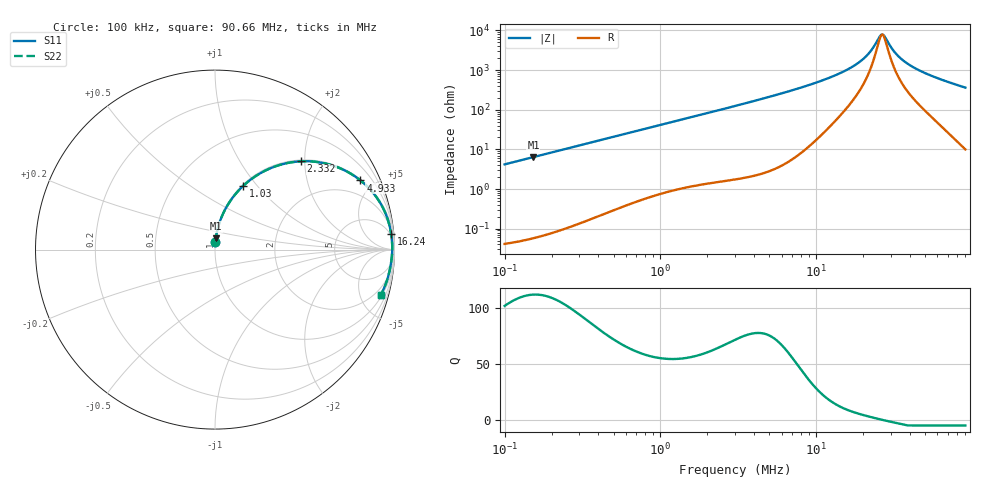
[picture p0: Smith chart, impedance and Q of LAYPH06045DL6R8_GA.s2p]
! LAYPH06045DL6R8_GA  S-PARAMETER MODEL  ( General Type )
! Model Generated by TAIYO YUDEN Corporation (http://www.ty-top.com)
! Version 2.0
! TAIYO YUDEN Control No. 180914NI43SB-FBB
! Copyright(c) 2018 TAIYO YUDEN CO.,LTD. All Rights Reserved.
! Product Description (link to TY-COMPAS)
! https://ds.yuden.co.jp/TYCOMPAS/or/detail?pn=LAYPH06045DL6R8NGA&u=M
! Products Name : Inductors
! Characteristics :
!  Inductance : 6.8 uH , SRF(min) : -Hz , DC Resistance(max) : 0.0377 Ohm
!  Rated Current : Saturation :2.5 A , Temp Rise : 2 A (25 degC)
!  Case Size : 6.3 x 6.0 / 0.248 x 0.236 [mm/inch] , Thickness : 4.5 / 0.177 [mm/inch]
!  (Conditions: Temperature = 25 degC , DC Bias Current/Voltage = 0A / 0V)
! External Node Assignments :
!  1  o---GGG---o  2
! GND o---------o GND
! Frequency Range : 0.1MHz  -  90.659724MHz  [ 402 STEP ]
# MHz S RI R 50
! Freq[MHz].  S11 Real  S11 Imag  S21 Real  S21 Imag  S12 Real  S12 Imag  S22 Real  S22 Imag
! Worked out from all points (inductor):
!   401 points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, 100 kHz to 90.66 MHz, reference 50 ohm
!   read as one part in series: L = 6.67 uH near 103.5 kHz
!   highest Q = 112 at 153.1 kHz (marker M1), where L = 6.67 uH
!   self-resonance near 26.16 MHz
!   S11 on the Smith chart (normalised r, x): 100 kHz: 1.00, +0.08; 1.03 MHz: 1.02, +0.85; 2.332 MHz: 1.03, +1.92; 4.933 MHz: 1.06, +4.18; 16.24 MHz: 4, +22; 90.66 MHz: 1.20, -7.24
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0.1  0.00216 0.0418  0.9978 -0.0418  0.9978 -0.0418  0.00216 0.0418
0.153052  0.00466 0.0638  0.9953 -0.0638  0.9953 -0.0638  0.00466 0.0638
0.312872  0.0182 0.1283  0.9818 -0.1283  0.9818 -0.1283  0.0182 0.1283
0.597477  0.0614 0.2326  0.9386 -0.2326  0.9386 -0.2326  0.0614 0.2326
0.97889  0.1455 0.3436  0.8545 -0.3436  0.8545 -0.3436  0.1455 0.3436
1.030183  0.1582 0.3559  0.8418 -0.3559  0.8418 -0.3559  0.1582 0.3559
1.523933  0.286 0.443  0.714 -0.443  0.714 -0.443  0.286 0.443
2.332406  0.4799 0.4918  0.5201 -0.4918  0.5201 -0.4918  0.4799 0.4918
3.062674  0.6143 0.4799  0.3857 -0.4799  0.3857 -0.4799  0.6143 0.4799
4.933098  0.8104 0.3854  0.1896 -0.3854  0.1896 -0.3854  0.8104 0.3854
9.420503  0.9465 0.2099  0.0535 -0.2099  0.0535 -0.2099  0.9465 0.2099
12.79846  0.9714 0.1374  0.0286 -0.1374  0.0286 -0.1374  0.9714 0.1374
16.24304  0.9812 0.0885  0.0188 -0.0885  0.0188 -0.0885  0.9812 0.0885
18.61296  0.9845 0.063  0.0155 -0.063  0.0155 -0.063  0.9845 0.063
20.96864  0.9864 0.0414  0.0136 -0.0414  0.0136 -0.0414  0.9864 0.0414
26.16292  0.9876 0.00253  0.0124 -0.00253  0.0124 -0.00253  0.9876 0.00253
27.53385  0.9874 -0.00635  0.0126 0.00635  0.0126 0.00635  0.9874 -0.00635
29.47413  0.9869 -0.0182  0.0131 0.0182  0.0131 0.0182  0.9869 -0.0182
34.35444  0.9847 -0.0449  0.0153 0.0449  0.0153 0.0449  0.9847 -0.0449
42.14104  0.9797 -0.0813  0.0203 0.0813  0.0203 0.0813  0.9797 -0.0813
58.23478  0.9662 -0.1449  0.0338 0.1449  0.0338 0.1449  0.9662 -0.1449
90.65972  0.9232 -0.2529  0.0768 0.2529  0.0768 0.2529  0.9232 -0.2529
